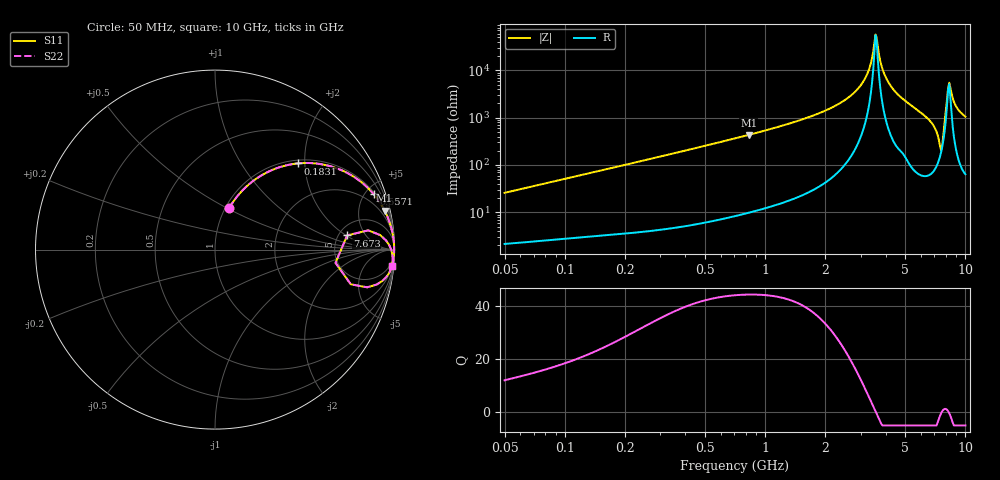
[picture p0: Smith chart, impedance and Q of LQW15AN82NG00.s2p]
!Murata Part Number: LQW15AN82NG00
!These Parameters are Measured in Series Mode Connection
!  o--[Z]--o
!Port1  Port2
!  o-------o
!Freq. Start=50[MHz] Stop=10[GHz], 401[Steps]
# Hz S RI R 50
!Freq.(Hz)	S 11(Real)	S 11(Imag)	S 21(Real)	S 21(Imag)	S 12(Real)	S 12(Imag)	S 22(Real)	S 22(Imag)
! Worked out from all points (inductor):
!   401 points, 50 MHz to 10 GHz, reference 50 ohm
!   read as one part in series: L = 81.5 nH near 51.34 MHz
!   highest Q = 44.2 at 828.9 MHz (marker M1), where L = 83.2 nH
!   self-resonance near 3.559 GHz
!   S11 on the Smith chart (normalised r, x): 50 MHz: 1.04, +0.51; 183.1 MHz: 1.07, +1.85; 557.1 MHz: 1.13, +5.68; 7.673 GHz: 5.96, +2.09; 10 GHz: 2, -21
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5e7  0.0794 0.2318  0.9206 -0.2318  0.9206 -0.2318  0.0794 0.2318
1.214486e8  0.2842 0.4275  0.7158 -0.4275  0.7158 -0.4275  0.2842 0.4275
1.831143e8  0.4618 0.4802  0.5382 -0.4802  0.5382 -0.4802  0.4618 0.4802
2.949953e8  0.6836 0.451  0.3164 -0.451  0.3164 -0.451  0.6836 0.451
5.57107e8  0.8841 0.3086  0.1159 -0.3086  0.1159 -0.3086  0.8841 0.3086
7.071068e8  0.9253 0.2518  0.0747 -0.2518  0.0747 -0.2518  0.9253 0.2518
8.289263e8  0.9451 0.2168  0.0549 -0.2168  0.0549 -0.2168  0.9451 0.2168
1.717543e9  0.9893 0.0905  0.0107 -0.0905  0.0107 -0.0905  0.9893 0.0905
2.917498e9  0.9977 0.0239  0.00227 -0.0239  0.00227 -0.0239  0.9977 0.0239
3.243629e9  0.9982 0.0115  0.0018 -0.0115  0.0018 -0.0115  0.9982 0.0115
3.558764e9  0.9983 0.000477  0.00168 -0.000477  0.00168 -0.000477  0.9983 0.000477
3.654301e9  0.9983 -0.0027  0.00169 0.0027  0.00169 0.0027  0.9983 -0.0027
3.904516e9  0.9981 -0.0108  0.00186 0.0108  0.00186 0.0108  0.9981 -0.0108
4.171863e9  0.9978 -0.0191  0.00224 0.0191  0.00224 0.0191  0.9978 -0.0191
6.54512e9  0.9817 -0.1054  0.0183 0.1054  0.0183 0.1054  0.9817 -0.1054
7.276762e9  0.9005 -0.1948  0.0995 0.1948  0.0995 0.1948  0.9005 -0.1948
7.472112e9  0.7566 -0.1934  0.2434 0.1934  0.2434 0.1934  0.7566 -0.1934
7.672705e9  0.7365 0.0791  0.2635 -0.0791  0.2635 -0.0791  0.7365 0.0791
8.090191e9  0.9694 0.0269  0.0306 -0.0269  0.0306 -0.0269  0.9694 0.0269
8.307378e9  0.9834 -0.0065  0.0166 0.0065  0.0166 0.0065  0.9834 -0.0065
9.114482e9  0.9897 -0.0622  0.0103 0.0622  0.0103 0.0622  0.9897 -0.0622
1e10  0.9855 -0.0928  0.0145 0.0928  0.0145 0.0928  0.9855 -0.0928
